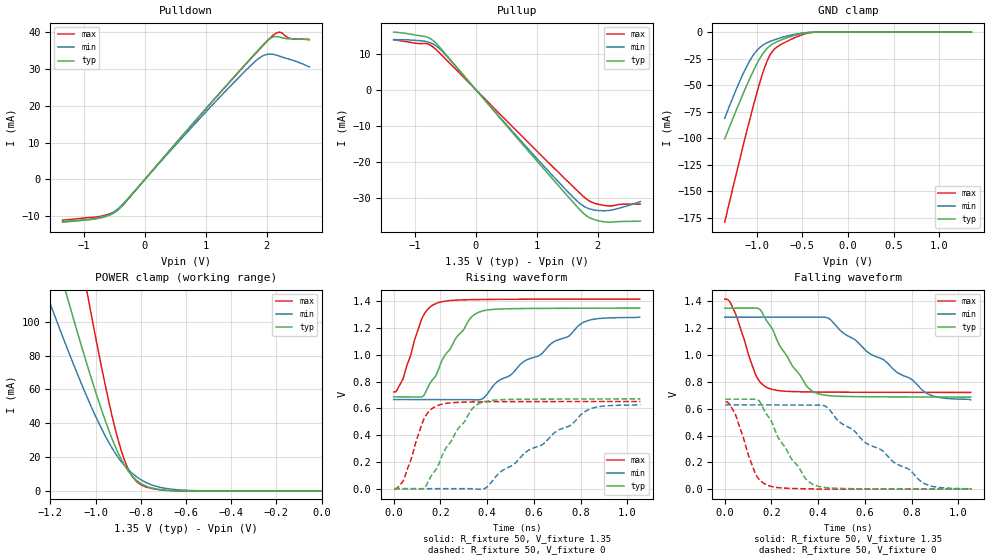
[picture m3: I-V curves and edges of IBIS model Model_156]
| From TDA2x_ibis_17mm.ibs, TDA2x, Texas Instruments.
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| Model based on original model for DDR_SEIOPB_V
|   Sub model SR101_DRV48_1P35
[model]   Model_156
|[Description]  [1.35V-I/O-X-X]
|   , ,
|[Input Load]
|[Output Drive]
|Voltage   1.35V
|Mode   I/O
Model_type   I/O
Polarity   Non-Inverting
Enable   Active-Low
Vinl =  0.585
Vinh =  0.765
Cref =  15.0000pF
Rref =  100.0000M
Vref =  0V
Vmeas =  0.675
C_comp   2p   2p   2p
[Model Spec]
Vinl   0.585   0.55125   0.61875
Vinh   0.765   0.73125   0.79875
[Receiver Thresholds]
Tslew_ac = 5n
Vth= 0.675
Vth_max= 0.709
Vth_min= 0.608
Vinh_ac= 0.175
Vinh_dc= 0.1
Vinl_ac= -0.175
Vinl_dc= -0.1
[Temperature Range]   25   125   -40
[Voltage Range]   1.35   1.2825   1.4175
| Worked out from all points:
|   slope of the pulldown table from 0 to 0.203 V, typ, clamps not added: 51.5 ohm
|   slope of the pullup table from 0 to 0.203 V, typ, clamps not added: 50.4 ohm
|   GND clamp passes 1 mA (typ) near -0.48 V on its own axis
|   POWER clamp passes 1 mA (typ) near -0.72 V on its own axis
|   rising waveform, R_fixture 50, V_fixture 1.35: 20-80 % time 139ps typ, 324ps min, 75.9ps max; typ from 0.687 V to 1.35 V
|   rising waveform, R_fixture 50, V_fixture 0: 20-80 % time 137ps typ, 318ps min, 74.3ps max; typ from 0 V to 0.671 V
|   falling waveform, R_fixture 50, V_fixture 1.35: 20-80 % time 137ps typ, 306ps min, 77.4ps max; typ from 1.35 V to 0.687 V
|   falling waveform, R_fixture 50, V_fixture 0: 20-80 % time 138ps typ, 312ps min, 74.3ps max; typ from 0.671 V to 0 V
[POWER_clamp]
-1.35V    224.4mA    165.8mA    358.5mA
-1.214V   157mA      115.5mA    250.8mA
-1.132V   117.8mA    86.59mA    187.7mA
-1.118V   111.4mA    81.92mA    177.3mA
-1.036V   74.26mA    55.16mA    116.8mA
-954.5mV  40.7mA     31.91mA    61.06mA
-900mV    22.42mA    19.79mA    30.14mA
-859.1mV  12.48mA    13.09mA    13.96mA
-804.5mV  4.85mA     7.084mA    4.132mA
-736.4mV  1.313mA    2.9mA      1.073mA
-627.3mV  101.6uA    577.3uA    45.9uA
0V        75.63nA    322.4nA    418.5nA
[Pulldown]
-1.35V    -11.61mA   -11.5mA    -11.06mA
-736.4mV  -10.48mA   -10.33mA   -10.03mA
-531.8mV  -9.35mA    -9.062mA   -9.043mA
-409.1mV  -7.817mA   -7.49mA    -7.751mA
1.145V    21.94mA    20.88mA    21.88mA
1.718V    32.55mA    30.62mA    32.41mA
1.923V    36.25mA    33.48mA    36.08mA
2.005V    37.61mA    33.98mA    37.53mA
2.086V    38.57mA    34.03mA    38.89mA
2.209V    38.7mA     33.51mA    40.04mA
2.373V    38.22mA    32.66mA    38.36mA
2.7V      37.95mA    30.56mA    38.05mA
[Pullup]
-1.35V    15.95mA    13.86mA    13.81mA
-981.8mV  15.11mA    13.66mA    12.86mA
-818.2mV  14.65mA    13.35mA    12.79mA
-736.4mV  14.02mA    12.92mA    12.23mA
-613.6mV  12.13mA    11.6mA     10.47mA
1.064V    -20.91mA   -20.19mA   -18.01mA
1.555V    -30.35mA   -29.03mA   -26.14mA
1.759V    -34.1mA    -32.12mA   -29.45mA
1.923V    -35.82mA   -33.22mA   -31.26mA
2.168V    -36.64mA   -33.43mA   -32.13mA
2.414V    -36.45mA   -32.48mA   -31.67mA
2.7V      -36.37mA   -30.94mA   -31.63mA
[GND_clamp]
-1.35V    -100.7mA   -81.27mA   -179.3mA
-1.241V   -77.31mA   -57.61mA   -140mA
-1.132V   -54.83mA   -36.31mA   -101.6mA
-1.05V    -39.08mA   -23.36mA   -74mA
-968.2mV  -25.28mA   -14.71mA   -48.34mA
-913.6mV  -18.13mA   -11.32mA   -33.52mA
-859.1mV  -13.28mA   -9.024mA   -22.35mA
-831.8mV  -11.61mA   -8.091mA   -18.64mA
-777.3mV  -9.078mA   -6.444mA   -14.07mA
-531.8mV  -1.871mA   -1.307mA   -3.441mA
-368.2mV  -88.76uA   -111.2uA   -158uA
1.35V     75.63nA    385.5nA    349.4nA
[Ramp]
dV/dt_f 0.39863622/0.13715036n 0.37089331/0.30694405n 0.41798725/77.535733p
dV/dt_r  0.4046726/0.13790153n 0.37920479/0.31964517n 0.39243793/74.510377p
R_load = 50
[Rising Waveform]
R_fixture = 50
V_fixture = 1.35
V_fixture_min = 1.2825
V_fixture_max = 1.4175
0s        686.6mV    666.1mV    722.5mV
39.28ps   685.9mV    666.1mV    817.7mV
125.1ps   690.2mV    666mV      1.287V
184.8ps   859.4mV    666.1mV    1.387V
268.5ps   1.13V      665.8mV    1.41V
330.9ps   1.279V     665mV      1.413V
372ps     1.324V     666.5mV    1.414V
552.9ps   1.347V     945.3mV    1.416V
811.6ps   1.349V     1.243V     1.417V
1.053ns   1.35V      1.282V     1.417V
[Rising Waveform]
R_fixture = 50
V_fixture = 0
V_fixture_min = 0
V_fixture_max = 0
3.075ps   0V         0V         0V
43.34ps   0V         0V         67.48mV
129.1ps   0V         0V         518.7mV
192.6ps   181.1mV    0V         624.6mV
273.6ps   442.9mV    0V         645.1mV
336.8ps   598.5mV    0V         648.4mV
378.2ps   645.3mV    -3.15mV    649.4mV
568.2ps   668.7mV    276.8mV    651.2mV
826.8ps   670.6mV    585.1mV    651.7mV
1.056ns   671.4mV    628.3mV    651.8mV
[Falling Waveform]
R_fixture = 50
V_fixture = 1.35
V_fixture_min = 1.2825
V_fixture_max = 1.4175
0s        1.35V      1.282V     1.417V
20.86ps   1.35V      1.283V     1.4V
48.83ps   1.35V      1.283V     1.299V
134.9ps   1.351V     1.283V     844.6mV
191.6ps   1.227V     1.283V     750.1mV
290ps     918.7mV    1.283V     728mV
394.8ps   715.3mV    1.284V     724.6mV
448.4ps   697.1mV    1.27V      723.7mV
866.5ps   687.5mV    713.5mV    721.9mV
1.053ns   686.6mV    666.1mV    721.8mV
[Falling Waveform]
R_fixture = 50
V_fixture = 0
V_fixture_min = 0
V_fixture_max = 0
3.075ps   671.4mV    628.3mV    650.9mV
46.59ps   671.6mV    628.3mV    553.5mV
131.8ps   671.1mV    628.4mV    115.1mV
185.8ps   542.6mV    628.3mV    27.59mV
285.6ps   227.2mV    628.3mV    5.187mV
388.2ps   28.36mV    628.6mV    0V
437.1ps   11.02mV    612.2mV    0V
598.3ps   2.591mV    352.4mV    0V
852.6ps   0V         43.39mV    0V
1.056ns   0V         0V         0V
